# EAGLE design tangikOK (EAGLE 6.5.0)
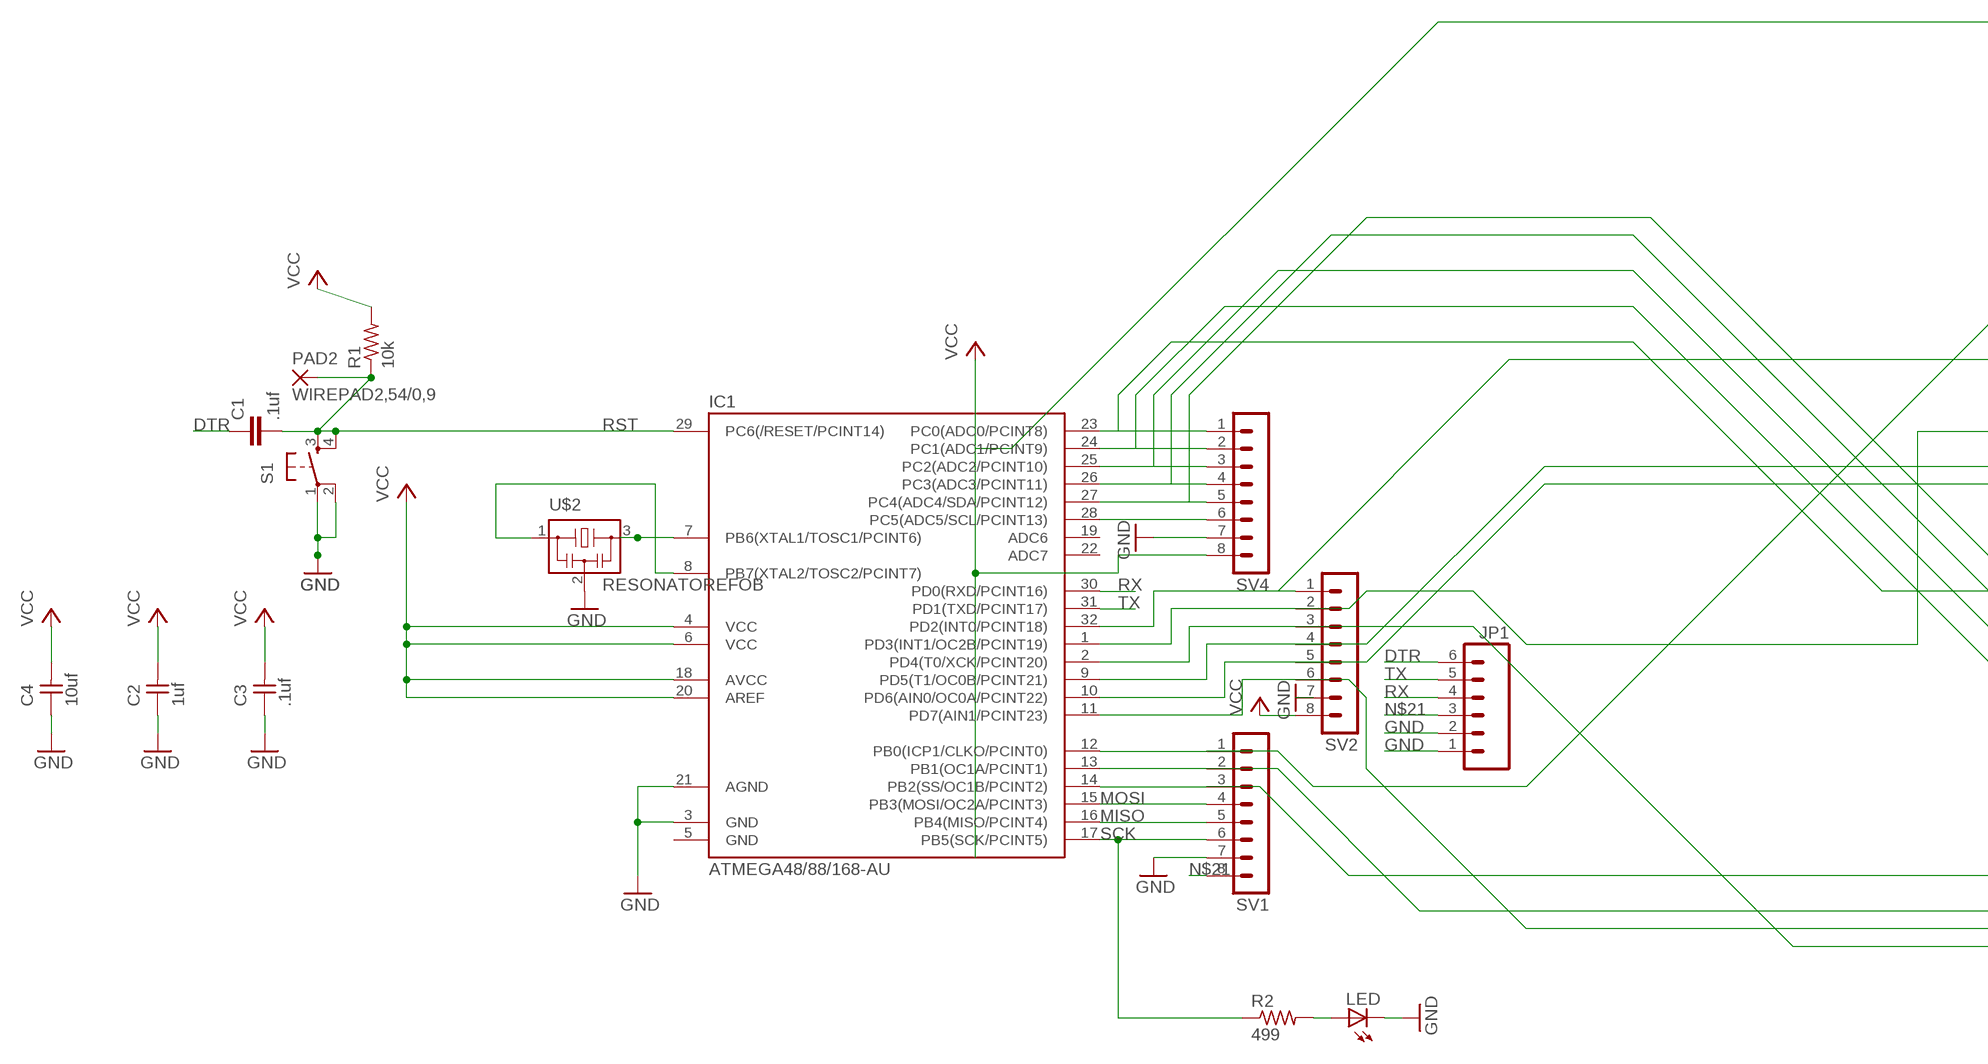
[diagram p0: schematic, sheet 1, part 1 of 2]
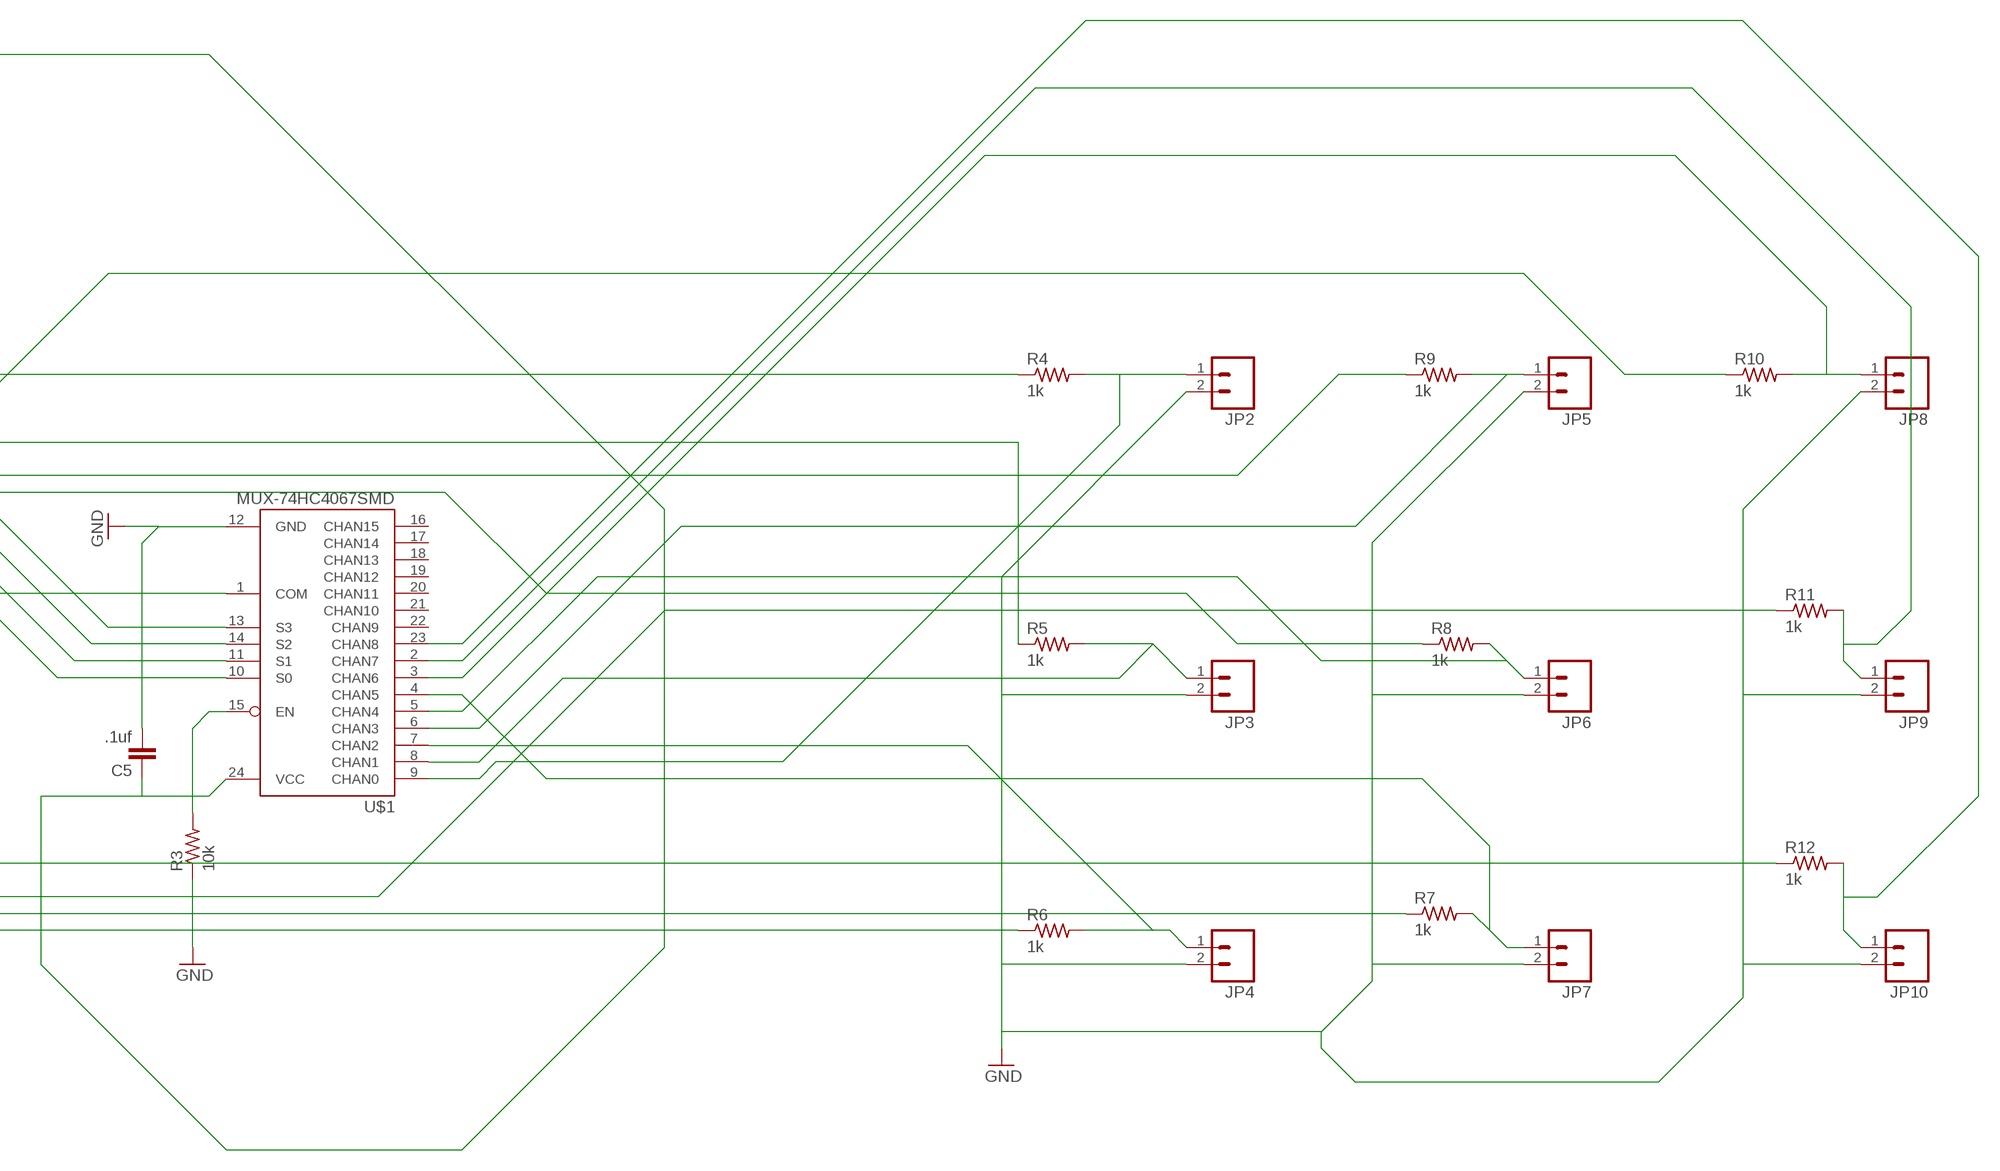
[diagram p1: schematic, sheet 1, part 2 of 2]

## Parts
C1  .1uf  C-EUC1206  [C1206]
C2  1uf  UNPOLARIZED_CAPACITOR1206  [1206]
C3  .1uf  UNPOLARIZED_CAPACITOR1206  [1206]
C4  10uf  UNPOLARIZED_CAPACITOR1206  [1206]
C5  .1uf  C-EUC1206  [C1206]
IC1  ATMEGA48/88/168-AU  [TQFP32-08]
JP1  M06SMD  [1X06-SMD]
JP2  M02  [1X02_LONGPADS]
JP3  M02  [1X02_LONGPADS]
JP4  M02  [1X02_LONGPADS]
JP5  M02  [1X02_LONGPADS]
JP6  M02  [1X02_LONGPADS]
JP7  M02  [1X02_LONGPADS]
JP8  M02  [1X02_LONGPADS]
JP9  M02  [1X02_LONGPADS]
JP10  M02  [1X02_LONGPADS]
LED  LED1206  [1206]
PAD2  WIREPAD2,54/0,9  [2,54/0,9]
R1  10k  RESISTOR1206  [1206]
R2  499  RESISTOR1206  [1206]
R3  10k  RESISTOR1206  [1206]
R4  1k  RESISTOR1206  [1206]
R5  1k  RESISTOR1206  [1206]
R6  1k  RESISTOR1206  [1206]
R7  1k  RESISTOR1206  [1206]
R8  1k  RESISTOR1206  [1206]
R9  1k  RESISTOR1206  [1206]
R10  1k  RESISTOR1206  [1206]
R11  1k  RESISTOR1206  [1206]
R12  1k  RESISTOR1206  [1206]
S1  6MM_SWITCH6MM_SWITCH  [6MM_SWITCH]
SV1  MA08-1  [MA08-1]
SV2  MA08-1  [MA08-1]
SV4  MA08-1  [MA08-1]
U$1  MUX-74HC4067SMD  [SSOP24]
U$2  RESONATOREFOB  [EFOBM]

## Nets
DTR: C1.1 JP1.6
GND: C2.1 C3.1 C4.1 C5.2 IC1.3(GND) IC1.21(AGND) JP1.1 JP1.2 JP2.2 JP3.2 JP4.2 JP5.2 JP6.2 JP7.2 JP8.2 JP9.2 JP10.2 LED.2(C) R3.1 S1.1(P) S1.2(P1) SV1.7 SV2.7 SV4.7 U$1.12(GND) U$2.2
MISO: IC1.16(PB4(MISO/PCINT4)) SV1.5
MOSI: IC1.15(PB3(MOSI/OC2A/PCINT3)) SV1.4
N$1: IC1.8(PB7(XTAL2/TOSC2/PCINT7)) U$2.1
N$2: IC1.12(PB0(ICP1/CLKO/PCINT0)) R10.1 SV1.1
N$4: IC1.24(PC1(ADC1/PCINT9)) SV4.2 U$1.10(S0)
N$5: IC1.25(PC2(ADC2/PCINT10)) SV4.3 U$1.11(S1)
N$7: IC1.27(PC4(ADC4/SDA/PCINT12)) SV4.5 U$1.13(S3)
N$8: IC1.28(PC5(ADC5/SCL/PCINT13)) SV4.6
N$9: IC1.7(PB6(XTAL1/TOSC1/PCINT6)) U$2.3
N$10: IC1.32(PD2(INT0/PCINT18)) R4.1 SV2.1
N$11: IC1.1(PD3(INT1/OC2B/PCINT19)) R5.1 SV2.2
N$12: IC1.2(PD4(T0/XCK/PCINT20)) R6.1 SV2.3
N$13: IC1.9(PD5(T1/OC0B/PCINT21)) R9.1 SV2.4
N$14: IC1.10(PD6(AIN0/OC0A/PCINT22)) R8.1 SV2.5
N$15: IC1.11(PD7(AIN1/PCINT23)) R7.1 SV2.6
N$17: IC1.13(PB1(OC1A/PCINT1)) R11.1 SV1.2
N$18: IC1.14(PB2(SS/OC1B/PCINT2)) R12.1 SV1.3
N$21: C2.2 C3.2 C4.2 C5.1 IC1.4(VCC) IC1.6(VCC) IC1.18(AVCC) IC1.20(AREF) JP1.3 R1.2 SV1.8 SV2.8 SV4.8 U$1.24(VCC) ; supply symbol labelled VCC
N$22: R3.2 U$1.15(EN)
N$23: LED.1(A) R2.2
N$24: IC1.23(PC0(ADC0/PCINT8)) SV4.1 U$1.1(COM)
N$26: IC1.26(PC3(ADC3/PCINT11)) SV4.4 U$1.14(S2)
N$29: JP4.1 R6.2 U$1.7(CHAN2)
N$30: JP3.1 R5.2 U$1.8(CHAN1)
N$31: JP2.1 R4.2 U$1.9(CHAN0)
N$32: JP5.1 R9.2 U$1.6(CHAN3)
N$33: JP6.1 R8.2 U$1.5(CHAN4)
N$34: JP8.1 R10.2 U$1.3(CHAN6)
N$35: JP9.1 R11.2 U$1.2(CHAN7)
N$36: JP10.1 R12.2 U$1.23(CHAN8)
N$37: JP7.1 R7.2 U$1.4(CHAN5)
RST: C1.2 IC1.29(PC6(/RESET/PCINT14)) PAD2.1(P) R1.1 S1.3(S) S1.4(S1)
RX: IC1.30(PD0(RXD/PCINT16)) JP1.4
SCK: IC1.17(PB5(SCK/PCINT5)) R2.1 SV1.6
TX: IC1.31(PD1(TXD/PCINT17)) JP1.5
Unconnected: IC1.19(ADC6) IC1.22(ADC7) U$1.16(CHAN15) U$1.17(CHAN14) U$1.18(CHAN13) U$1.19(CHAN12) U$1.20(CHAN11) U$1.21(CHAN10) U$1.22(CHAN9)

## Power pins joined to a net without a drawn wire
GND: IC1.5(GND)

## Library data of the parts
C1 C5 = rcl:C-EU: CAPACITOR, European symbol
C2-C4 = ng:UNPOLARIZED_CAPACITOR: unpolarized_capacitor
IC1 = atmega8:ATMEGA48/88/168
JP1 = SparkFun:M06: Header 6 Standard 6-pin 0.1" header. Use with straight break away headers (SKU : PRT-00116), right angle break away headers (PRT-00553), swiss pins (PRT-00743), machine pins (PRT-00117), and female headers (PRT-00115). Molex polarized connector foot print use with SKU : PRT-08094 with associated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
JP2-JP10 = 01_SparkFun:M02: Header 2
LED = ng:LED
PAD2 = wirepad:WIREPAD: Wire PAD connect wire on PCB
R1-R12 = ng:RESISTOR
S1 = ng:6MM_SWITCH: OMRON SWITCH
SV1 SV2 SV4 = con-lstb:MA08-1: PIN HEADER
U$1 = 01_SparkFun:MUX-74HC4067
U$2 = fab:RESONATOR

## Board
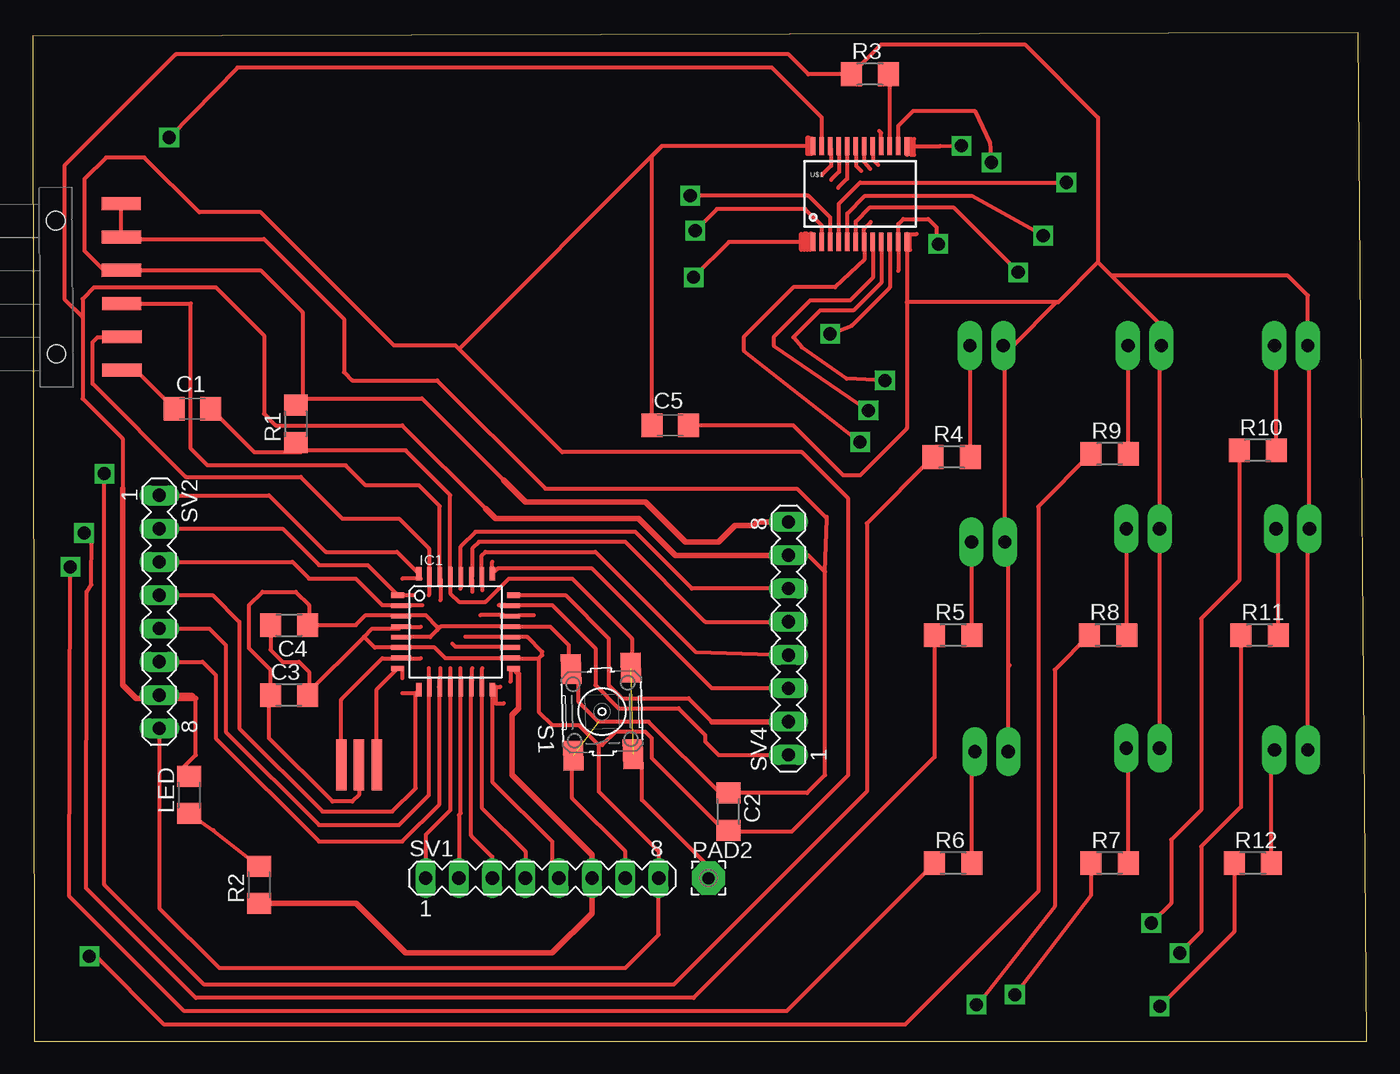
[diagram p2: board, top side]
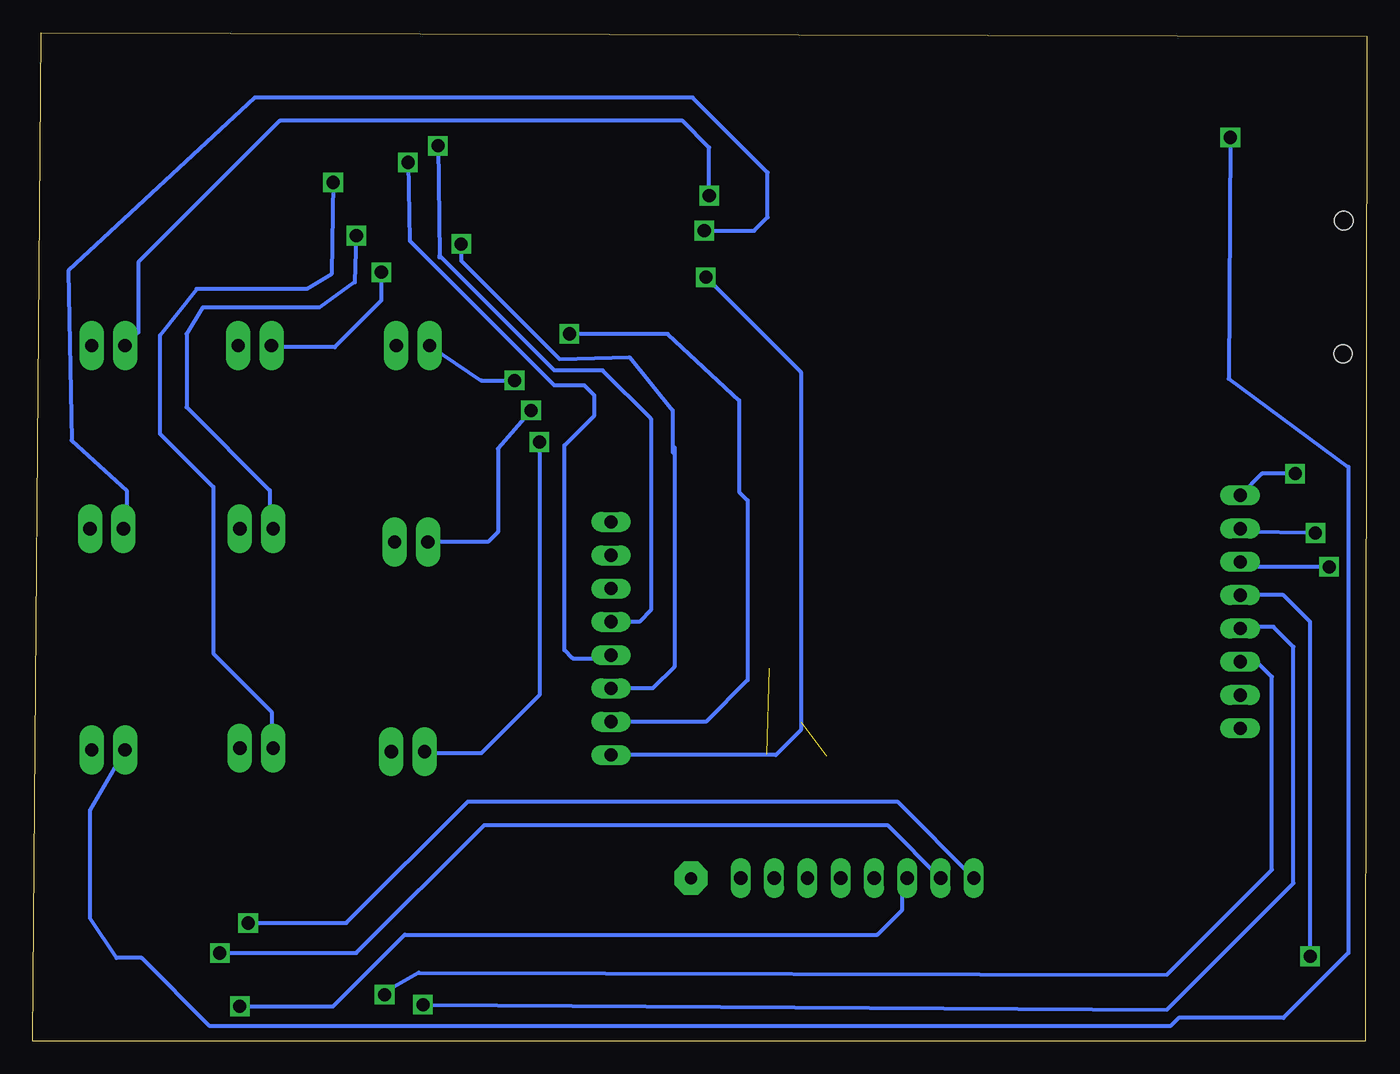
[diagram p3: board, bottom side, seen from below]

Size 101.78 x 76.95 mm. Coordinates in mm from the lower left corner, seen from the top.
Outline: 0.13,0 101.78,0 101.14,76.95 0,76.7 0.13,0
Copper layers (1*16): Top 0.035mm / dielectric 1.5mm / Bottom 0.035mm
Design rules "default": minimum track width 10mil, minimum drill 24mil, track to track 8mil, track to pad 8mil, pad to pad 8mil, via to via 8mil, smd to smd 8mil, copper to edge 40mil, drill to drill 8mil, minimum pad ring 10mil, minimum via ring 8mil, stop-mask expansion 4mil, vias tented up to drill 0mil, thermal gap 10mil

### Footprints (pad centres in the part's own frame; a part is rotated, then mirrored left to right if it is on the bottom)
C1206 = smd 1.6 x 1.8: 1 -1.4,0; 2 1.4,0
1206 = smd 1.6 x 1.803: 1 -1.422,0; 2 1.422,0
TQFP32-08 = smd 1.016 x 0.406: 1 -4.42,2.8; 8 -4.42,-2.8; 17 4.42,-2.8; 24 4.42,2.8 | smd 1.524 x 0.356: 2 -4.166,2; 3 -4.166,1.2; 4 -4.166,0.4; 5 -4.166,-0.4; 6 -4.166,-1.2; 7 -4.166,-2; 18 4.166,-2; 19 4.166,-1.2; 20 4.166,-0.4; 21 4.166,0.4; 22 4.166,1.2; 23 4.166,2 | smd 0.406 x 1.016: 9 -2.8,-4.42; 16 2.8,-4.42; 25 2.8,4.42; 32 -2.8,4.42 | smd 0.356 x 1.524: 10 -2,-4.166; 11 -1.2,-4.166; 12 -0.4,-4.166; 13 0.4,-4.166; 14 1.2,-4.166; 15 2,-4.166; 26 2,4.166; 27 1.2,4.166; 28 0.4,4.166; 29 -0.4,4.166; 30 -1.2,4.166; 31 -2,4.166
1X06-SMD = smd 1 x 3: 1 -6.35,5; 2 -3.81,5; 3 -1.27,5; 4 1.27,5; 5 3.81,5; 6 6.35,5 | hole 1.4: -5.08,0; 5.08,0
1X02_LONGPADS = drill 1.016 pad 1.88 long: 1 0,0; 2 2.54,0
2,54/0,9 = drill 0.914 pad 2.54 octagon: 1 0,0
6MM_SWITCH = smd 2.286 x 1.524: 1 -3.302,2.286; 2 3.302,2.286; 3 -3.302,-2.286; 4 3.302,-2.286
MA08-1 = drill 1.016 long: 1 -8.89,0; 2 -6.35,0; 3 -3.81,0; 4 -1.27,0; 5 1.27,0; 6 3.81,0; 7 6.35,0; 8 8.89,0
SSOP24 = smd 0.348 x 1.397: 1 -3.575,-3.656; 2 -2.925,-3.656; 3 -2.275,-3.656; 4 -1.625,-3.656; 5 -0.975,-3.656; 6 -0.325,-3.656; 7 0.325,-3.656; 8 0.975,-3.656; 9 1.625,-3.656; 10 2.275,-3.656; 11 2.925,-3.656; 12 3.575,-3.656; 13 3.575,3.656; 14 2.925,3.656; 15 2.275,3.656; 16 1.625,3.656; 17 0.975,3.656; 18 0.325,3.656; 19 -0.325,3.656; 20 -0.975,3.656; 21 -1.625,3.656; 22 -2.275,3.656; 23 -2.925,3.656; 24 -3.575,3.656
EFOBM = smd 0.8 x 3.9: 1 -1.35,0; 2 0,0; 3 1.35,0

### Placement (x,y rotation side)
C1  12.19,48.26 0 top
C2  53.09,17.53 270 top
C3  19.56,26.42 0 top
C4  19.56,31.75 180 top
C5  48.64,46.99 0 top
IC1  32.26,31.24 0 top
JP1  1.78,57.53 270.3 top
JP2  71.5,53.09 0 top
JP3  71.63,38.1 0 top
JP4  71.88,22.1 0 top
JP5  83.57,53.09 0 top
JP6  83.44,39.12 0 top
JP7  83.44,22.35 0 top
JP8  94.74,53.09 0 top
JP9  94.87,39.12 0 top
JP10  94.74,22.22 0 top
LED  11.94,18.8 90 top
PAD2  51.56,12.45 0 top
R1  20.07,47.12 90 top
R2  17.27,11.94 90 top
R3  63.88,73.79 0 top
R4  70.1,44.58 0 top
R5  70.23,30.99 0 top
R6  70.23,13.59 0 top
R7  82.17,13.59 0 top
R8  82.04,30.99 0 top
R9  82.17,44.83 0 top
R10  93.47,45.09 0 top
R11  93.6,30.99 0 top
R12  93.09,13.59 0 top
S1  43.43,25.15 91.5 top
SV1  38.86,12.45 0 top
SV2  9.65,32.77 270 top
SV4  57.66,30.73 90 top
U$1  63.12,64.64 0 top
U$2  24.89,21.08 180 top

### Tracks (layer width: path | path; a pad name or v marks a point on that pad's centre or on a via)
DTR
  Top 0.305: C1.1 7.85,51.21 JP1.6
GND  (1 unrouted)
  Top 0.305: JP1.2 JP1.1 | U$2.2 24.89,18.8 24.38,18.29 22.86,18.29 18.03,23.11 18.03,26.31 C3.1 18.14,28.35 16.51,29.97 16.51,33.27 17.53,34.29 20.07,34.29 21.08,33.27 21.08,31.85 C4.1 24.64,31.75 25.4,32.51 28.02,32.51 IC1.3 28.16,32.51 29.97,32.51 30.86,31.62 30.86,31.37 | LED.2 11.18,20.57 12.45,21.84 12.45,26.16 12.19,26.42 SV2.7 | 30.86,31.37 31.13,31.64 IC1.21 39.48,31.64 40.89,30.23 40.89,28.55 S1.2 41.66,27.79 41.66,25.91 43.18,24.38 46.99,24.38 52.43,18.95 C2.1 59.08,18.95 60.45,20.32 60.45,35.81 | 30.86,31.37 30.33,30.84 IC1.5 | SV1.7 45.21,14.48 41.15,18.54 41.15,21.7 S1.1 | 60.45,35.81 59.18,37.08 SV4.7 | 60.45,35.81 60.58,39.89 | 60.58,39.89 60.58,40.01 | 3.81,55.25 3.81,56.64 4.7,57.53 13.97,57.53 17.65,53.85 17.65,47.88 18.54,46.99 28.19,46.99 34.54,40.64 | 3.81,55.25 3.81,49.02 6.86,45.97 6.86,41.66 | 6.91,61.21 17.65,61.21 23.75,55.12 23.75,51.05 24.38,50.42 30.86,50.42 39.12,42.16 58.3,42.16 60.58,39.89 | 3.81,55.25 2.41,56.64 2.41,66.8 10.92,75.31 57.66,75.31 59.18,73.79 R3.1 64.75,76.07 75.69,76.07 81.28,70.48 81.28,59.44 | U$1.12 66.69,56.39 | 66.69,56.39 66.69,46.76 63.12,43.18 61.85,43.18 58.04,46.99 50.55,46.99 50.29,46.99 | 50.29,46.99 50.04,46.74 | 81.28,59.44 78.23,56.39 78.11,56.39 | 78.11,56.39 66.69,56.39 | 78.11,56.39 74.8,53.09 JP2.2 74.17,52.96 JP3.2 74.42,37.85 74.42,28.57 | JP4.2 74.42,28.57 | 82.3,58.42 86.11,54.61 JP5.2 85.98,52.96 JP7.2 JP6.2 | 74.55,28.7 74.42,28.57 | 82.3,58.42 95.76,58.42 97.28,56.9 JP8.2 97.41,52.96 JP9.2 97.28,38.99 JP10.2 | 82.3,58.42 81.28,59.44 | C5.2 50.29,46.99
  Top 0.406: 12.45,26.16 7.87,26.16 6.86,27.18 6.86,41.66 6.86,42.16 | 34.54,40.64 35.31,39.88 46.23,39.88 49.02,37.08 SV4.7 | 6.91,61.21 JP1.2
MISO
  Top 0.305: IC1.16 35.06,19.81 39.62,15.24 39.62,12.95 SV1.5 39.67,11.98
MOSI
  Top 0.305: IC1.15 34.26,17.81 37.59,14.48 SV1.4
N$1
  Top 0.305: U$2.1 26.24,26.85 IC1.8
N$2  (via drill 0.6, 1)
  Top 0.305: IC1.12 31.86,17.63 29.97,15.75 SV1.1 | R10.1 92.05,35.15 89.15,32.26 89.15,17.65 86.87,15.37 86.87,10.54 v85.34,9.02
  Bottom 0.305: v85.34,9.02 77.85,9.02 68.58,18.29 35.81,18.29 SV1.1
N$3
  Top 0.305: 66.68,61.6 67.44,61.6
N$4  (via drill 1)
  Top 0.305: IC1.24 40.64,34.04 43.94,30.73 43.94,27.18 44.96,26.16 50.04,26.16 51.82,24.38 | U$1.10 65.39,57.52 62.48,54.61 v60.83,53.98
  Top 0.406: 51.82,24.38 SV4.2
  Bottom 0.305: SV4.2 50.42,24.38 47.24,27.56 47.24,41.28 47.88,41.91 47.88,48.9 53.34,53.98 v60.83,53.98
N$5  (via drill 1)
  Top 0.305: SV4.3 51.82,26.92 42.67,36.07 35.46,36.07 IC1.25 | U$1.11 66.04,62.36 66.42,62.74 68.33,62.74 68.96,62.1 68.96,60.96 v69.09,60.83
  Bottom 0.305: 52.83,45.34 52.83,44.83 | 52.83,44.83 52.83,28.57 54.48,26.92 SV4.3 | 52.83,44.83 52.96,44.96 52.96,48.13 56.26,52.2 61.59,52.07 69.09,59.56 v69.09,60.83
N$6
  Top 0.305: 66.04,60.71 66.04,58.8
N$7  (via drill 0.6, 1)
  Top 0.305: IC1.27 33.53,35.48 33.53,37.59 34.04,38.1 45.21,38.1 51.31,32 SV4.5 | U$1.13 69.24,68.3 v70.87,68.33
  Bottom 0.305: v70.87,68.33 70.74,59.94 | 70.74,59.94 70.74,59.82 | SV4.5 55.5,32 54.61,32.89 54.61,47.5 58.29,51.18 61.98,51.18 70.74,59.94
N$8
  Top 0.305: SV4.6 50.29,34.54 45.97,38.86 33.78,38.86 32.66,37.74 IC1.28
N$9
  Top 0.305: U$2.3 23.54,26.08 26.67,29.21 28.06,29.21 IC1.7
N$10  (via drill 0.6, 1)
  Top 0.305: SV2.1 18.03,41.66 22.35,37.34 27.78,37.34 IC1.32 | R4.1 63.63,39.52 63.63,19.05 48.89,4.32 13.08,4.32 5.46,11.94 v5.46,43.18 v5.46,43.31
  Bottom 0.305: v5.46,43.31 8,43.31 SV2.1
N$11  (via drill 1)
  Top 0.305: SV2.2 19.05,39.12 21.84,36.32 25.56,36.32 IC1.1 | R5.1 68.81,21.69 50.42,3.3 12.45,3.3 4.06,11.68 4.12,34.29 4.47,34.85 4.5,38.58 v3.91,38.79
  Bottom 0.305: v3.91,38.79 9.4,38.86 SV2.2
N$12  (via drill 1)
  Top 0.305: SV2.3 19.81,36.58 21.08,35.31 24.64,35.31 26.67,33.27 28.06,33.27 IC1.2 | R6.1 57.51,2.29 11.56,2.29 2.79,11.05 v2.87,36.2
  Bottom 0.305: v2.87,36.2 9.27,36.2 SV2.3
N$13  (via drill 0.6, 1)
  Top 0.305: SV2.4 13.72,34.04 15.75,32 15.75,23.88 22.1,17.53 27.43,17.53 29.21,19.3 29.21,26.57 IC1.9 | R9.1 76.71,40.79 76.71,11.43 66.55,1.27 10.03,1.27 4.83,6.48 v4.32,6.48
  Bottom 0.305: v4.32,6.48 4.32,32 6.35,34.04 SV2.4
N$14  (via drill 1)
  Top 0.305: SV2.5 13.46,31.5 14.73,30.23 14.73,23.62 21.84,16.51 27.94,16.51 30.23,18.8 30.23,27.04 IC1.10 | R8.1 77.98,28.35 77.98,10.29 72.39,3.17 v72.01,2.79
  Bottom 0.305: v72.01,2.79 15.24,2.41 5.59,12.07 5.59,30.1 7.11,31.62 9.53,31.62 SV2.5
N$15  (via drill 0.6, 1)
  Top 0.305: SV2.6 12.95,28.96 13.97,27.94 13.97,23.11 21.84,15.24 28.19,15.24 30.99,18.03 30.99,27.01 IC1.11 | R7.1 80.75,11.15 v74.93,3.56
  Bottom 0.305: SV2.6 8.38,28.96 7.24,27.81 7.24,13.08 15.24,5.08 72.34,5.23 74.75,3.83 74.8,3.68 v74.93,3.56
N$16
  Top 0.305: 6.73,58.93 6.48,58.67
N$17  (via drill 0.6, 1)
  Top 0.305: IC1.13 32.66,17.42 32.51,17.27 SV1.2 | R11.1 92.18,17.88 89.15,14.86 89.15,8.38 v87.5,6.73
  Bottom 0.305: v87.5,6.73 77.09,6.73 67.31,16.51 36.58,16.51 SV1.2
N$18  (via drill 0.6, 1)
  Top 0.305: IC1.14 33.46,15.68 35.05,14.08 SV1.3 | R12.1 91.67,8.36 v85.98,2.67
  Bottom 0.305: v85.98,2.67 78.87,2.67 73.41,8.13 37.34,8.13 35.43,10.03 35.43,12.07 SV1.3
N$19
  Top 0.305: 63.42,61.24 63.42,62 63.93,62.51
N$20
  Top 0.305: 59.46,61.62 59.31,61.62 59.31,60.4 59.08,60.4 59.08,61.62 58.85,61.62 58.85,60.4 58.62,60.4 58.62,61.62
N$21
  Top 0.305: 25.27,30.86 20.98,26.57 C3.2 21.08,26.52 21.08,28.19 20.32,28.96 19.05,28.96 18.14,29.87 C4.2 | 25.27,30.86 25.91,31.5 27.95,31.5 IC1.4 | 25.27,30.86 26.09,30.04 IC1.6 30.66,30.04 31.5,29.21 36.39,29.21 IC1.18 36.46,29.21 38.61,29.21 | 9.4,23.88 SV2.8 9.65,10.16 14.22,5.59 45.21,5.59 47.75,8.13 SV1.8 47.75,14.48 43.18,19.05 43.18,22.61 | 38.61,29.21 38.86,29.46 38.86,29.72 37.74,30.84 IC1.20 | 38.61,29.21 38.61,25.15 39.62,24.13 41.66,24.13 43.18,22.61 | 43.18,22.61 43.43,22.61 44.45,23.62 46.74,23.62 47.24,23.11 47.24,21.59 52.83,16 53.09,16 | 53.09,16 57.91,16 62.23,20.32 62.23,41.4 58.67,44.96 40.39,44.96 32.51,52.83 | 20.57,49.05 20.57,55.63 17.37,58.83 JP1.3 6.49,58.55 5.71,58.55 3.94,60.33 3.94,65.79 5.59,67.44 8.51,67.44 12.7,63.25 17.4,63.25 27.56,53.09 32.26,53.09 32.51,52.83 | 20.57,49.05 R1.2 | 20.57,49.05 29.69,49.05 35.92,42.82 | U$1.24 48.01,68.3 | 48.01,68.3 47.98,68.3 32.51,52.83 | C5.1 47.24,67.53 48.01,68.3 | C2.2 53.09,16
  Top 0.406: SV4.8 55.27,39.62 55.02,39.37 53.59,39.37 52.32,38.1 49.78,38.1 46.74,41.15 37.59,41.15 35.92,42.82
N$22
  Top 0.305: U$1.15 65.39,73.04 65.28,73.15 65.28,73.76 R3.2
N$23
  Top 0.305: LED.1 13.77,16.1 R2.2
N$24  (via drill 0.6, 1)
  Top 0.305: IC1.23 36.46,33.27 39.62,33.27 42.93,29.97 42.93,27.18 44.7,25.4 49.28,25.4 51.31,23.37 51.31,22.86 52.32,21.84 SV4.1 | U$1.1 53.11,60.99 v50.42,58.29
  Bottom 0.305: v50.42,58.29 43.18,51.05 43.18,23.75 45.09,21.84 SV4.1
N$25
  Top 0.305: 59.54,68.86 59.38,68.86 59.38,67.72 59.23,67.72 59.23,68.94 59.08,68.94 59.08,67.72
N$26  (via drill 0.6, 1)
  Top 0.305: IC1.26 34.26,37.05 34.54,37.34 42.93,37.34 50.55,29.72 SV4.4 | U$1.14 66.04,69.85 67.18,70.99 71.88,70.99 73.03,68.58 v73.15,67.06
  Bottom 0.305: v73.15,67.06 73.03,61.09 61.98,50.04 59.69,50.04 58.93,49.28 58.93,47.75 61.21,45.47 61.21,29.84 60.58,29.21 57.91,29.21 SV4.4
N$27
  Top 0.305: 60.91,68.1 60.91,66.8 60.22,66.12
N$28
  Top 0.305: 61.52,68.1 61.52,66.34 60.91,65.73
N$29  (via drill 0.6, 1)
  Top 0.305: R6.2 71.65,21.87 JP4.1 | U$1.7 63.44,59.63 61.21,57.53 58.04,57.53 54.23,53.72 54.23,52.71 v63.12,45.72
  Bottom 0.305: v63.12,45.72 63.12,26.42 67.56,21.97 71.76,21.97 JP4.1
N$30  (via drill 1)
  Top 0.305: R5.2 71.65,38.08 JP3.1 | U$1.8 64.09,58.25 62.36,56.52 59.31,56.52 56.52,53.72 56.52,53.09 v63.75,48.13
  Bottom 0.305: v63.75,48.13 66.29,45.21 66.29,38.86 67.06,38.1 JP3.1
N$31  (via drill 1)
  Top 0.305: R4.2 71.53,53.06 JP2.1 | U$1.9 64.74,57.89 62.61,55.75 60.07,55.75 58.04,53.72 58.67,52.96 62.1,50.55 v65.02,50.42
  Bottom 0.305: JP2.1 67.56,50.42 v65.02,50.42
N$32  (via drill 0.6, 1)
  Top 0.305: R9.2 83.59,53.06 JP5.1 | U$1.6 62.79,62.54 63.88,63.63 70.23,63.63 v75.18,58.67
  Bottom 0.305: v75.18,58.67 75.18,56.52 78.74,52.96 83.44,52.96 JP5.1
N$33  (via drill 0.6, 1)
  Top 0.305: R8.2 83.46,39.09 JP6.1 | U$1.5 62.14,63.16 63.5,64.52 71.63,64.52 v77.09,61.47
  Bottom 0.305: v77.09,61.47 77.22,57.91 79.91,55.98 88.8,55.98 90.04,53.98 90.04,48.39 83.69,42.04 83.69,39.37 JP6.1
N$34  (via drill 0.6, 1)
  Top 0.305: R10.2 94.89,52.93 JP8.1 | U$1.3 60.84,62.85 59.18,64.52 v50.16,64.52
  Bottom 0.305: v50.16,64.52 50.16,68.2 52.2,70.23 82.93,70.23 93.73,59.44 93.73,54.1 JP8.1
N$35  (via drill 0.6, 1)
  Top 0.305: R11.2 95.02,39.01 95.38,39.37 95.12,39.37 JP9.1 | U$1.2 60.19,62.23 58.93,63.5 52.2,63.5 v50.55,61.85
  Bottom 0.305: v50.55,61.85 46.74,61.85 45.72,62.87 45.72,66.29 51.43,72.01 84.84,72.01 99.06,58.8 98.81,45.85 94.62,42.04 94.62,39.37 JP9.1
N$36  (via drill 1)
  Top 0.305: R12.2 94.51,22 JP10.1 | U$1.23 60.19,70.49 56.39,74.3 15.62,74.3 v10.41,68.96
  Bottom 0.305: v10.41,68.96 10.54,50.55 1.4,43.82 1.4,6.73 6.35,1.78 14.35,1.78 14.99,1.14 88.27,1.14 93.47,6.35 95.38,6.35 97.41,9.4 97.41,17.65 JP10.1
N$37  (via drill 0.6, 1)
  Top 0.305: R7.2 83.59,22.2 JP7.1 | U$1.4 61.49,63.91 63.12,65.53 v78.87,65.53
  Bottom 0.305: v78.87,65.53 78.99,58.55 80.9,57.4 89.28,57.4 92.08,53.85 92.08,46.36 88.01,42.29 88.01,29.59 83.57,25.15 83.57,22.48 JP7.1
N$38
  Top 0.305: 62.13,68.02 62.13,65.81 61.44,65.13
N$39
  Top 0.305: 62.81,67.79 62.81,66.8 63.2,66.42
N$40
  Top 0.305: 63.42,68.4 63.42,67.11 63.88,66.57
N$41
  Top 0.305: 64.11,67.64 64.11,67.26 64.49,66.88
N$42
  Top 0.305: 36.07,30.86 33.02,30.86
N$43
  Top 0.305: 36.2,30.1 32.26,30.1 32,30.35
N$44
  Top 0.305: 36.45,28.45 36.45,27.43
N$45
  Top 0.305: 35.05,27.05 35.31,27.05 | 35.31,27.05 35.31,25.78 35.94,25.78 | 35.31,27.05 35.69,27.05
N$46
  Top 0.305: 34.29,27.69 34.29,28.45
N$47
  Top 0.305: 33.53,27.56 33.53,28.45
N$48
  Top 0.305: 32.64,27.43 32.64,28.45
N$49
  Top 0.305: 31.88,27.43 31.88,28.45
N$50
  Top 0.305: 31.12,27.3 31.12,28.45
N$51
  Top 0.305: 30.23,27.43 30.23,28.45
N$52
  Top 0.305: 29.46,26.54 28.19,26.54
N$53
  Top 0.305: 28.19,28.45 28.19,27.69
N$54
  Top 0.305: 28.7,29.21 29.59,29.21
N$55
  Top 0.305: 28.58,31.62 29.59,31.62
N$56
  Top 0.305: 28.45,33.27 29.72,33.27
N$57
  Top 0.305: 28.19,34.04 29.08,34.04
N$58
  Top 0.305: 29.59,35.31 28.19,35.31
N$59
  Top 0.305: 30.23,35.31 30.23,34.04
N$60
  Top 0.305: 31.12,35.31 31.12,33.66
N$61
  Top 0.305: 32.64,35.18 32.64,34.54
N$62
  Top 0.305: 33.53,35.18 33.53,34.29
N$63
  Top 0.305: 34.29,35.18 34.29,34.42
N$64
  Top 0.305: 35.05,35.81 35.05,36.58
N$65
  Top 0.305: 37.08,32.51 38.23,32.51
N$66
  Top 0.305: 35.94,32.51 34.16,32.51
N$67
  Top 0.305: 36.07,33.27 35.56,33.27
N$68
  Top 0.305: 64.72,68.86 64.72,69.32 64.57,69.47
N$69
  Top 0.305: 66.7,67.64 66.7,68.86 67.01,68.86 67.01,67.64 67.23,67.64 67.23,68.86
N$70
  Top 0.305: 66.78,60.4 66.93,60.4 66.93,61.54
RST  (1 unrouted)
  Top 0.305: C1.2 16.89,44.96 20.45,44.96 20.07,45.34 R1.1 20.68,45.09 28.45,45.09 31.86,41.68 IC1.29 31.86,34.18 32.51,33.53 34.54,33.53 36.32,35.31 41.15,35.31 45.72,30.73 45.72,28.59 S1.4 45.59,28.45 | PAD2.1 51.56,13.34 46.48,18.41 46.48,21.23 S1.3
RX
  Top 0.305: IC1.30 31.06,40.82 29.46,42.42 25.4,42.42 23.88,43.94 13.33,43.94 12.06,45.21 12.06,56.29 JP1.4
SCK
  Top 0.406: R2.1 24.66,10.52 28.45,6.73 39.62,6.73 42.67,9.78 SV1.6 42.67,14.22 36.58,20.32 36.58,24.89 37.08,25.4 37.08,28.04 IC1.17
TX
  Top 0.305: IC1.31 30.23,35.44 30.23,37.59 27.94,39.88 23.62,39.88 20.45,43.05 11.68,43.05 4.57,50.16 4.57,53.34 4.95,53.72 6.77,53.72 JP1.5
